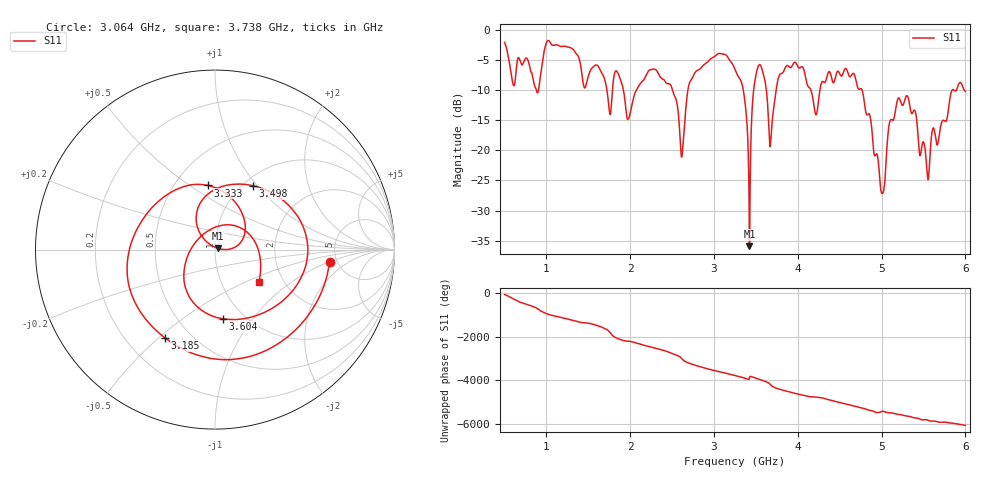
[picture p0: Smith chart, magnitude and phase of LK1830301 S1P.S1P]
!Agilent Technologies,E5071C,
!Date:
!Data & Calibration Information:
!Freq	S11:SOLT1(ON)
!PortZ  Port1:50+j0
!Above PortZ is port z conversion or system Z0 setting when saving the data.
!When reading, reference impedance value at option line is always used.
# Hz S dB R 50
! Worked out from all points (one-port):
!   1601 points, 500 MHz to 6 GHz, reference 50 ohm
!   lowest |S11| = -35.9 dB at 3.422 GHz (marker M1), VSWR 1.03, Z = 51.4 + j0.761 ohm
!   |S11| at or under -10 dB: 1.918 GHz to 2.071 GHz (152.9 MHz wide, 7.66 % of centre); 2.505 GHz to 2.687 GHz (182.1 MHz wide, 7.02 % of centre); 4.767 GHz to 5.841 GHz (1.073 GHz wide, 20.2 % of centre)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
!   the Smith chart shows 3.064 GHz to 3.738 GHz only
!   S11 on the Smith chart (normalised r, x): 3.064 GHz: 4.34, -0.99; 3.185 GHz: 0.36, -0.52; 3.333 GHz: 0.72, +0.59; 3.498 GHz: 1.11, +0.95; 3.604 GHz: 0.80, -0.73; 3.738 GHz: 1.50, -0.61
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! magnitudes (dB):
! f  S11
! 500 MHz  -2.0
! 885 MHz  -10.3
! 1.005 GHz  -1.9
! 1.188 GHz  -2.7
! 1.755 GHz  -13.8
! 1.875 GHz  -7.9
! 1.975 GHz  -14.8
! 2.26 GHz  -6.5
! 2.562 GHz  -12.6
! 2.618 GHz  -20.9
! 2.721 GHz  -8.4
! 3.064 GHz  -3.9
! 3.185 GHz  -5.0
! 3.25 GHz  -6.5
! 3.333 GHz  -8.9
! 3.422 GHz  -35.9
! 3.498 GHz  -7.7
! 3.604 GHz  -8.2
! 3.673 GHz  -19.2
! 3.738 GHz  -10.3
! 3.938 GHz  -5.8
! 4.216 GHz  -14.1
! 4.625 GHz  -7.8
! 5.01 GHz  -27.2
! 5.103 GHz  -15.0
! 5.312 GHz  -11.1
! 5.553 GHz  -24.9
! 6 GHz  -10.1
